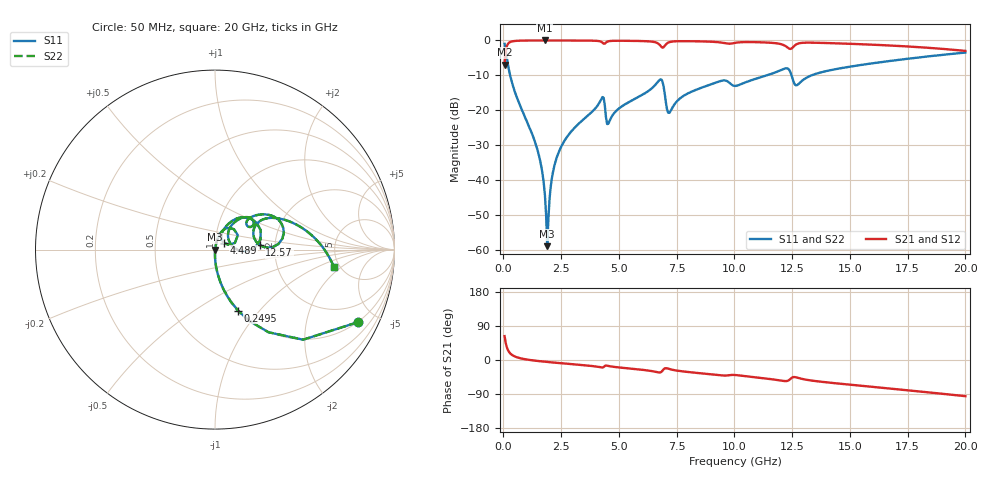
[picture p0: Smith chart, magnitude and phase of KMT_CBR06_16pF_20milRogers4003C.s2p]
! Data measured by Modelithics Inc. support@modelithics.com 813-866-6335
! KEMET CBR0603 16pF, Pad Width= 0.851mm, Pad Length= 0.64mm, Pad Gap= 0.62mm, 20mil Rogers 4003C substrate Data, January 2022
# hz S ma R 50
! 2 Port Network Data from SP1.SP block
! freq  magS11  angS11  magS21  angS21  magS12  angS12  magS22  angS22
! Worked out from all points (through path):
!   401 points, 50 MHz to 20 GHz, reference 50 ohm
!   highest |S21| = -0.01 dB at 1.796 GHz (marker M1); lowest = -6.9 dB at 50 MHz (marker M2)
!   group delay of S21, straight-line fit = 13.7 ps
!   lowest |S11| = -58.9 dB at 1.895 GHz (marker M3), VSWR 1.00, Z = 50.1 - j0.0332 ohm
!   |S11| at or under -10 dB: 290 MHz to 11.4 GHz (11.11 GHz wide, 190 % of centre); 12.47 GHz to 13.34 GHz (865.1 MHz wide, 6.7 % of centre)
!   |S22| runs from -58.9 to -1.0 dB; largest |S21 - S12| = 0
!   S11 on the Smith chart (normalised r, x): 50 MHz: 0.99, -3.93; 249.5 MHz: 0.99, -0.78; 4.489 GHz: 1.11, +0.08; 12.57 GHz: 1.66, +0.09; 20 GHz: 4.47, -1.59
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5e7  0.892 -27.0  0.4517 63.0  0.4517 63.0  0.892 -27.0
2.495e8  0.3626 -69.3  0.9314 20.6  0.9314 20.6  0.3626 -69.3
6.485e8  0.1336 -83.8  0.9904 5.9  0.9904 5.9  0.1336 -83.8
1.496375e9  0.02538 -90.4  0.9986 -2.6  0.9986 -2.6  0.02538 -90.4
1.695875e9  0.01206 -88.9  0.9988 -3.9  0.9988 -3.9  0.01206 -88.9
1.795625e9  0.006062 -84.3  0.9988 -4.5  0.9988 -4.5  0.006062 -84.3
1.895375e9  0.001136 -16.9  0.9988 -5.1  0.9988 -5.1  0.001136 -16.9
1.995125e9  0.005358 71.9  0.9988 -5.7  0.9988 -5.7  0.005358 71.9
2.14475e9  0.01308 78.2  0.9986 -6.6  0.9986 -6.6  0.01308 78.2
2.34425e9  0.02287 79.1  0.9984 -7.7  0.9984 -7.7  0.02287 79.1
3.391625e9  0.07057 75.1  0.9954 -13.3  0.9954 -13.3  0.07057 75.1
4.2395e9  0.1456 56.2  0.9541 -19.6  0.9541 -19.6  0.1456 56.2
4.488875e9  0.06357 35.3  0.958 -15.0  0.958 -15.0  0.06357 35.3
6.73325e9  0.2669 39.0  0.8843 -32.9  0.8843 -32.9  0.2669 39.0
7.182125e9  0.09197 31.8  0.9449 -23.8  0.9449 -23.8  0.09197 31.8
8.429e9  0.2019 53.2  0.9706 -34.4  0.9706 -34.4  0.2019 53.2
1.0025e10  0.2231 36.6  0.9227 -39.6  0.9227 -39.6  0.2231 36.6
1.22195e10  0.3983 20.7  0.8278 -55.7  0.8278 -55.7  0.3983 20.7
1.256862e10  0.2511 5.5  0.8207 -45.0  0.8207 -45.0  0.2511 5.5
1.336662e10  0.319 32.1  0.9282 -54.5  0.9282 -54.5  0.319 32.1
1.670825e10  0.5069 13.1  0.8466 -75.2  0.8466 -75.2  0.5069 13.1
2e10  0.6702 -8.4  0.7074 -95.4  0.7074 -95.4  0.6702 -8.4
